{attribute 'qualified_only'}
{attribute 'strict'}
TYPE E_PMLUnitMode :
(
	UNDEFINED		:=  0,
	AUTOMATIC		:=  1,
	MAINTENANCE 	:=  2,
	MANUAL 			:=  3,
	SEMIAUTOMATIC	:=  4,
	DRYRUN			:=  5,
	USERMODE1		:=  6,
	USERMODE2		:=  7,
	IDLE 			:=  8,
	ESTOP 			:=  9
);
END_TYPE
